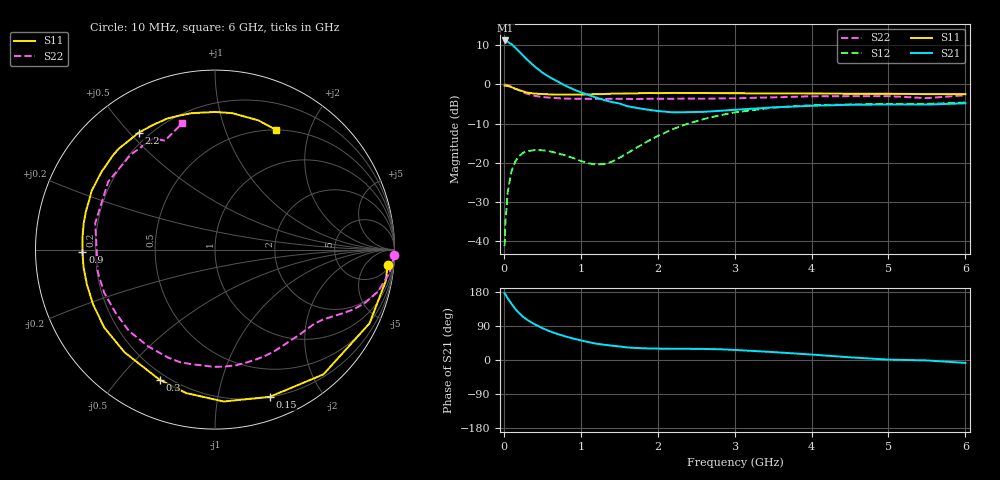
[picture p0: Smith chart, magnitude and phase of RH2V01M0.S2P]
! SIEMENS Small Signal Semiconductors
! BFR106
! Si NPN RF Bipolar Junction Transistor in SOT23
! VCE = 2 V  IC = 1 mA
! Common Emitter S-Parameters:  August  1996
# GHz  S  MA  R  50
!  f  S11  S21  S12  S22
! GHz  MAG  ANG  MAG  ANG  MAG  ANG  MAG  ANG
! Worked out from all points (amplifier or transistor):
!   36 points, 10 MHz to 6 GHz, reference 50 ohm
!   highest |S21| = 11.2 dB at 20 MHz (marker M1)
!   |S21| within 3 dB of that: start of sweep to 208.4 MHz
!   unconditionally stable (mu >= 1): 853.4 MHz to end of sweep
!   at 250 MHz: K = 0.28, MSG = 12.4 dB, |S12| = -17.4 dB
!   at 1.4 GHz: K = 1.50, MAG = 3.5 dB, |S12| = -19.7 dB
!   at 6 GHz: K = 1.02, MAG = -1.0 dB, |S12| = -4.6 dB
!   S11 on the Smith chart (normalised r, x): 10 MHz: 8, -19; 150 MHz: 0.20, -1.42; 300 MHz: 0.17, -0.65; 900 MHz: 0.15, -0.01; 2.2 GHz: 0.16, +0.53; 6 GHz: 0.50, +1.51
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0.01  0.9656 -5.1  3.6 176.0  0.0087 88.3  0.9999 -1.7
0.02  0.9676 -10.4  3.625 173.4  0.017 84.3  0.9955 -3.2
0.05  0.954 -25.5  3.488 162.7  0.0423 74.6  0.9793 -7.8
0.1  0.9211 -49.0  3.245 148.4  0.0784 62.6  0.9373 -14.5
0.15  0.8751 -69.6  2.926 134.1  0.1048 50.8  0.8836 -19.9
0.2  0.8477 -86.7  2.617 123.7  0.1225 42.5  0.8371 -23.6
0.25  0.8152 -101.4  2.33 113.9  0.1342 35.0  0.7933 -26.6
0.3  0.788 -113.1  2.079 106.5  0.1404 30.1  0.7618 -29.0
0.4  0.7625 -131.3  1.694 94.3  0.1457 21.7  0.7159 -33.0
0.5  0.7547 -144.8  1.414 84.1  0.1448 16.4  0.6902 -36.8
0.7  0.7397 -164.8  1.088 68.6  0.1327 11.3  0.6678 -45.3
0.9  0.7385 -178.8  0.868 56.7  0.1155 13.2  0.6558 -54.1
1.1  0.7461 168.7  0.732 47.2  0.099 22.4  0.6547 -64.2
1.3  0.7527 158.9  0.634 40.4  0.0969 39.9  0.6529 -74.5
1.6  0.7664 145.6  0.529 33.2  0.1317 61.9  0.6536 -90.5
2.2  0.7779 123.2  0.44 29.6  0.2694 64.6  0.6552 -124.6
2.8  0.7724 104.6  0.46 28.4  0.4022 50.4  0.6625 -158.8
3.5  0.7669 90.0  0.509 20.9  0.5063 32.5  0.6834 167.5
4.5  0.7589 76.8  0.55 7.1  0.5552 11.8  0.7076 131.7
5  0.7595 71.6  0.555 1.0  0.562 4.4  0.7081 119.0
5.5  0.7513 66.5  0.553 -1.1  0.5653 0.9  0.6683 114.7
6  0.7489 63.1  0.574 -7.7  0.5868 -6.5  0.7264 104.7
